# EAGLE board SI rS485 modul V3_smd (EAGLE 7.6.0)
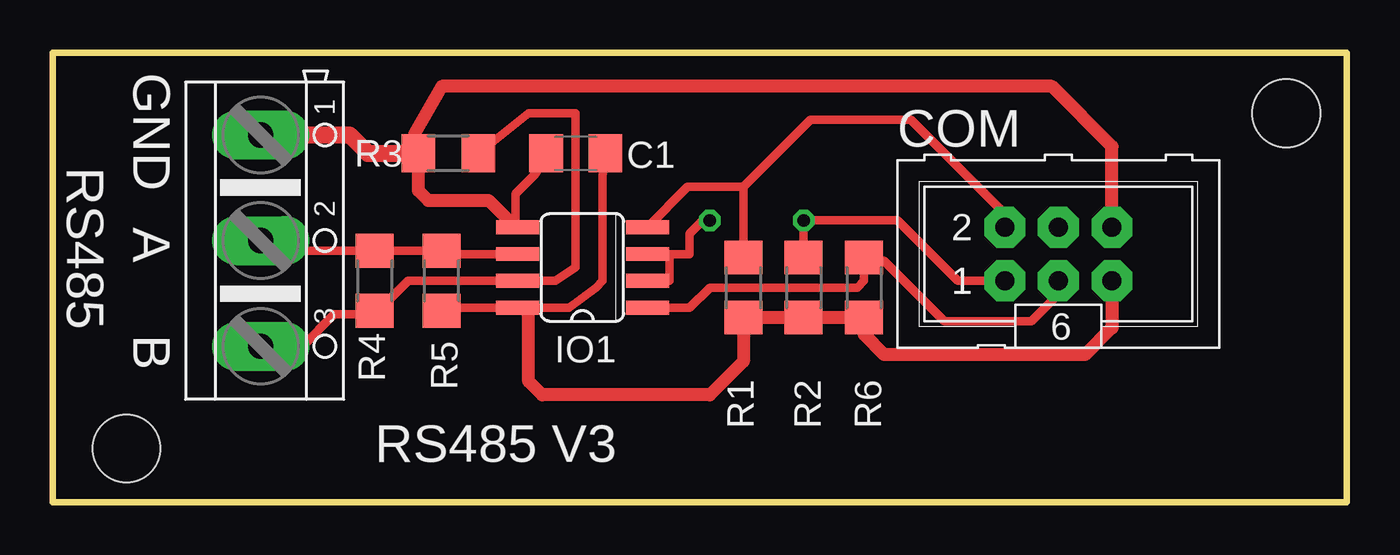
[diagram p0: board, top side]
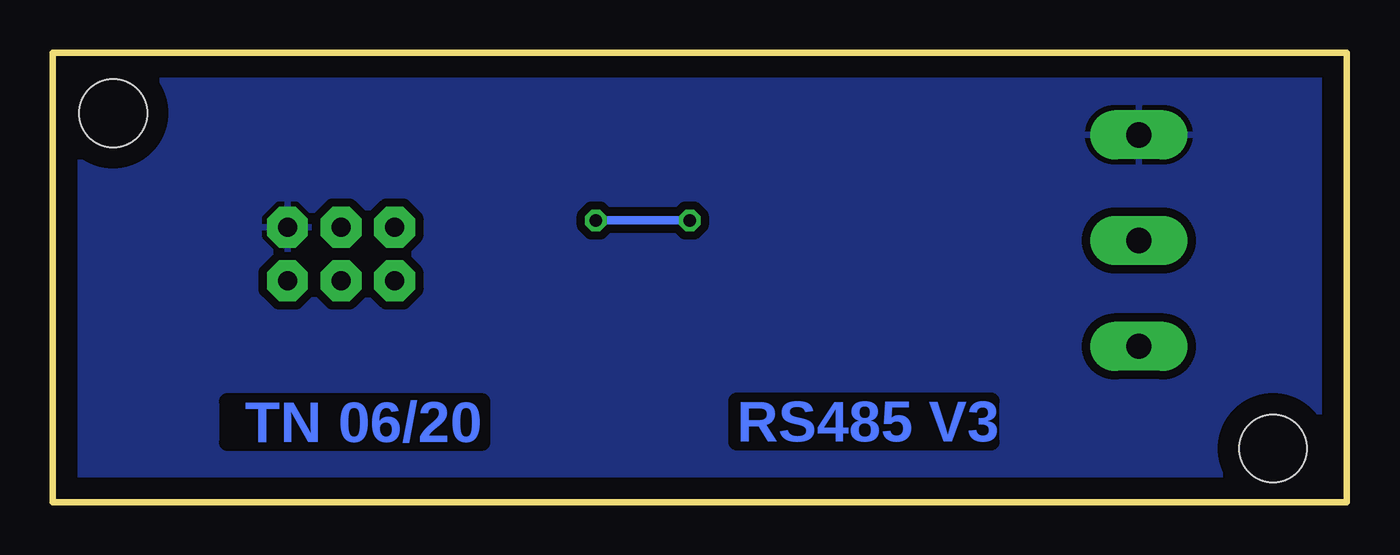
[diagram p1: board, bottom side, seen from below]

Size 61.28 x 21.27 mm. Coordinates in mm from the lower left corner, seen from the top.
Outline: 0,21.27 61.28,21.27 61.28,0 0,0 0,21.27
Copper layers (1*16): Top 0.035mm / dielectric 1.5mm / Bottom 0.035mm
Design rules "default": minimum track width 10mil, minimum drill 24mil, track to track 8mil, track to pad 8mil, pad to pad 8mil, via to via 8mil, smd to smd 8mil, copper to edge 40mil, drill to drill 8mil, minimum pad ring 10mil, minimum via ring 8mil, stop-mask expansion 4mil, vias tented up to drill 0mil, thermal gap 10mil
Holes 3.2 mm at 58.42,18.41 3.49,2.54

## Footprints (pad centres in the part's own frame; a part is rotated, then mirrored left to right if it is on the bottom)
C1206 = smd 1.6 x 1.8: 1 -1.4,0; 2 1.4,0
ML6 = drill 0.9 pad 1.93 octagon: 1 -2.54,-1.27; 2 -2.54,1.27; 3 0,-1.27; 4 0,1.27; 5 2.54,-1.27; 6 2.54,1.27
SO08 = smd 0.66 x 2.032: 1 -1.905,-3.073; 2 -0.635,-3.073; 3 0.635,-3.073; 4 1.905,-3.073; 5 1.905,3.073; 6 0.635,3.073; 7 -0.635,3.073; 8 -1.905,3.073
R1206 = smd 1.6 x 1.803: 1 -1.422,0; 2 1.422,0
AK500/3 = drill 1.2 pad 2.311 long: 1 -5.004,0; 2 0,0; 3 5.004,0

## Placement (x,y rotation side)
C1  100n  [C1206]  24.77,16.51 180 top
COM  [ML6]  47.62,11.75 0 top
IO1  MAX485  [SO08]  25.08,11.11 90 top
R1  10k  [R1206]  32.7,10.16 90 top
R2  10k  [R1206]  35.56,10.16 90 top
R3  20k  [R1206]  18.73,16.51 0 top
R4  120  [R1206]  15.24,10.48 90 top
R5  20k  [R1206]  18.41,10.48 270 top
R6  10k  [R1206]  38.42,10.16 90 top
RS485  [AK500/3]  9.84,12.38 270 top

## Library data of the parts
C1 R1-R6 = rcl
COM RS485 = 11moje
IO1 = maxim

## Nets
GND: C1.2 COM.6 IO1.5 R3.1 RS485.1
S$1: C1.1 COM.5 IO1.8 R1.1 R2.1 R5.2 R6.1
S$5: COM.1 IO1.2 IO1.3 R2.2
S$7: IO1.6 R4.2 R5.1 RS485.2
S$10: IO1.7 R3.2 R4.1 RS485.3
S$13: COM.3 IO1.1 R6.2
S$16: COM.2 IO1.4 R1.2

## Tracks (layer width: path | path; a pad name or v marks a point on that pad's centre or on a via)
GND
  Top 0.406: C1.2 22.86,15.56 21.91,14.61 21.91,13.12 IO1.5
  Top 0.61: COM.6 50.16,16.83 47.31,19.68 18.41,19.68 17.14,17.46 R3.1 17.31,14.76 17.78,14.29 20.64,14.29 21.59,13.34 21.69,13.34 IO1.5
  Top 0.813: RS485.1 14.05,17.39 14.92,16.51 R3.1
  pour Bottom (isolate 0.406): 0,21.27 61.28,21.27 61.28,0.32 0,0.32
S$1
  Top 0.406: R5.2 19.05,9.21 IO1.8 22.54,9.21 24.45,9.21 25.72,10.16 26.04,10.48 26.04,15.43 C1.1 | 38.42,7.94 R6.1
  Top 0.61: R6.1 R2.1 R1.1 32.7,6.67 31.11,5.08 23.18,5.08 22.54,5.71 22.54,9.21 | COM.5 50.16,8.26 48.9,6.99 39.37,6.99 38.42,7.94
S$5  (via drill 0.6)
  Top 0.406: R2.2 v35.56,13.34 40.01,13.34 42.86,10.48 COM.1 | v31.11,13.34 30.8,13.34 30.16,12.7 30.16,11.75 29.21,11.75 | 29.21,11.75 29.21,10.48 IO1.2 | 29.21,11.75 IO1.3
  Bottom 0.406: v31.11,13.34 v35.56,13.34
S$7
  Top 0.406: IO1.6 18.57,11.75 R5.1 R4.2 10.32,11.9 RS485.2
S$10
  Top 0.406: RS485.3 11.82,7.38 13.34,8.89 15.07,8.89 R4.1 15.4,9.06 16.83,10.48 IO1.7 23.81,10.48 24.77,11.11 24.77,18.41 22.54,18.41 R3.2
S$13
  Top 0.406: COM.3 47.62,9.84 46.35,8.57 42.23,8.57 39.37,11.43 38.57,11.43 R6.2 38.42,10.48 38.1,10.16 31.11,10.16 30.16,9.21 IO1.1
S$16
  Top 0.406: COM.2 45.09,13.65 40.64,18.1 35.88,18.1 32.7,14.92 | 32.7,14.92 R1.2 | 32.7,14.92 30.06,14.92 IO1.4

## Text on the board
Bottom: TN 06/20 | RS485 V3
tNames: GND | A | B | RS485 V3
